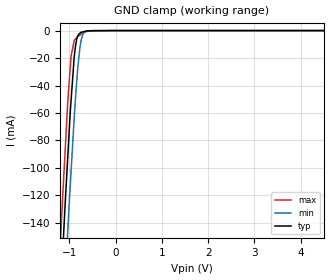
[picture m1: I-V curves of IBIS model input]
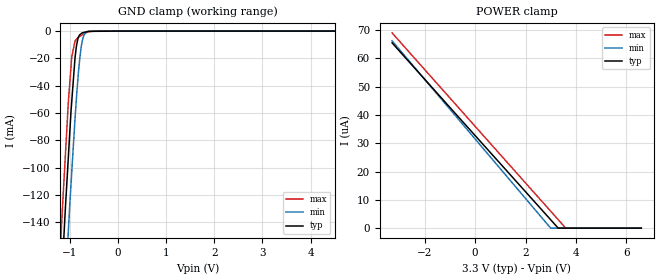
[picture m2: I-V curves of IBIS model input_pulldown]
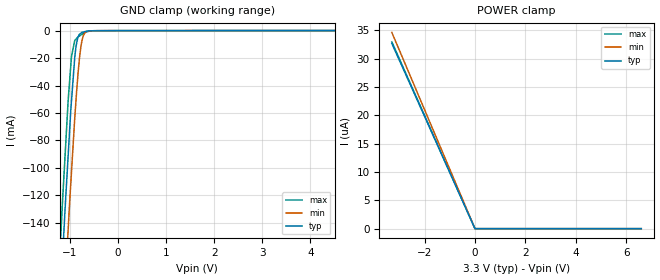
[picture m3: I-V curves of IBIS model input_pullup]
|Texas Instruments Incorporated
| Ultra-Small, Integrated Analog Front-End for Heart Rate Monitors and
| Low-Cost Pulse Oximeters
| Marketing part#   Digital Voltage Range   Package-type   #pins
| AFE4403   2.0V-3.6V   WCSP   36
[IBIS Ver]   4.1
[File name]   afe4403.ibs
[File Rev]   1.0
[Date]   6/3/2014
[Source]
| Texas Instruments Incorporated.
| Analog-eLab Design Center, HPA
| 12500 TI Blvd
| Dallas, TX -75243
[Notes]   Revision History:
| Rev 1.0: 6/3/2014
| - Initial version of the model
| - Model generated from simulations in TISPICE
| - Model matched to SPICE simulation
| - C_comp although listed in numerical order of value are
|   obtained from varying PVT conditions. For PVT conditions for
|   each specific value refer the buffer description under
|   respective [Model]. IBIS model user is responsible for using
|   appropriate C_comp to simulate for Signal Integrity.
| - All the models except io are taken from available IBIS model of AFE4490.
|*   EXCEPTION:   *
|*   - For input_pulldown and io models,there will be small leakage currents  *
|*   in POWER Clamp IV table because of a pulldown resistor R0 is connected *
|*   to PAD.   *
|*   - For model input_pullup,there will be  small leakage currents in GND   *
|*   Clamp IV table because of a pullup resistor R0 is connected to PAD.   *
[Disclaimer]
| This model is designed as an aid for customers of Texas Instruments.
| TI and its licensors and suppliers make no warranties, either expressed
| or implied, with respect to this  model, including the warranties of
| merchantability or fitness for a particular purpose. The model is
| provided solely on an "as is" basis. The entire risk as to its quality
| and performance is with the customer.
[Copyright]
(C) Copyright 2014 Texas Instruments Incorporated.All rights reserved.
|   AFE4403
[Component]   AFE4403
[Manufacturer]   TI
[Package]   |36 WCSP package
|   typ   min   max
R_pkg   0.01   0.008   0.12
L_pkg   0.1nH   0.08nH   0.12nH
C_pkg   0.1pF   0.08pF   0.12pF
[Pin]  signal_name   model_name   R_pin   L_pin   C_pin
A1   DNC   nc   na   na   na
A2   TX_CTRL_SUP   power   na   na   na
A3   LED_DRV_GND   gnd   na   na   na
A4   TXN   nc   na   na   na
A5   TXP   nc   na   na   na
A6   LED_DRV_SUP   power   na   na   na
B1   TX_REF   nc   na   na   na
B2   RX_DIG_GND   gnd   na   na   na
B3   TX3   nc   na   na   na
B4   DIAG_END   outp   na   na   na
B5   TG_EN   nc   na   na   na
B6   TG_OUT   io   na   na   na
C1   DNC   nc   na   na   na
C2   BG   nc   na   na   na
C3   AFE_PDN   input   na   na   na
C4   SPISIMO   outp   na   na   na
C5   SPISOMI   input_pulldown   na   na   na
C6   SCLK   input_pulldown   na   na   na
D1   VCM   nc   na   na   na
D2   VSS   gnd   na   na   na
D3   DNC   nc   na   na   na
D4   _RESET   input_pullup   na   na   na
D5   ADC_RDY   outp   na   na   na
D6   SPISTE   input_pullup   na   na   na
E1   INP   nc   na   na   na
E2   RX_ANA_GND   gnd   na   na   na
E3   DNC   nc   na   na   na
E4   RX_ANA_SUP   power   na   na   na
E5   RX_DIG_SUP   power   na   na   na
E6   CLKOUT   outp   na   na   na
F1   INN   nc   na   na   na
F2   RX_ANA_SUP   power   na   na   na
F3   XIN   nc   na   na   na
F4   XOUT   nc   na   na   na
F5   DNC   nc   na   na   na
F6   RX_DIG_GND   gnd   na   na   na
| Models and submodels in the file (5): input (Input), input_pulldown (Input), input_pullup (Input), outp (Output), io (I/O)
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|   input Model
[Model]   input
Model_type   Input
Vinl = 0.66
Vinh = 2.64
|   typ   min   max
|   (nom PVT)   (fast PVT)   (slow PVT)
C_comp   3.312e-13   3.289e-13   3.358e-13
[Model spec]
|subparameter
Vinl   0.66   0.6   0.72
Vinh   2.64   2.4   2.88
| Where nom  PVT is Nominal Process, 3.3V, 27C
|   Fast PVT is Strong Process,  3.6V, -40C
|   Slow PVT is Weak Process,   3V, 105C
[Voltage Range]   3.3   3   3.6
|Junction Temperature
[Temperature Range]   27   105   -40
[Power Clamp Reference]   3.3   3   3.6
[GND Clamp Reference]   0   0   0
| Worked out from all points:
|   GND clamp passes 1 mA (typ) near -0.72 V on its own axis
[GND Clamp]
|   Voltage   I(typ)   I(min)   I(max)
-3.3V     -1.734A    -1.762A    -1.725A
-1.27V    -245.7mA   -302.2mA   -207.4mA
-1.156V   -168.6mA   -223.4mA   -127.4mA
-1.137V   -156.2mA   -210.7mA   -115.7mA
-1.099V   -130.6mA   -186.4mA   -91.68mA
-1.037V   -92.87mA   -146.8mA   -52.56mA
-964.8mV  -51.35mA   -103.1mA   -18.88mA
-897.6mV  -19.84mA   -64.25mA   -7.375mA
-825mV    -4.345mA   -29.78mA   -4.502mA
-745.8mV  -1.232mA   -7.144mA   -2.676mA
-591mV    -190.8uA   -137.2uA   -416.9uA
6.6V      0A         0A         0A
[POWER Clamp]
|   Voltage   I(typ)   I(min)   I(max)
-3.3V     0A         0A         0A
0V        0A         0A         0A
6.6V      0A         0A         0A
|   input_pulldown Model
[Model]   input_pulldown
Model_type   Input
Vinl = 0.66
Vinh = 2.64
|   typ   min   max
|   (nom PVT)   (fast PVT)   (slow PVT)
C_comp   3.312e-13   3.289e-13   3.358e-13
[Model spec]
|subparameter
Vinl   0.66   0.6   0.72
Vinh   2.64   2.4   2.88
| Where nom  PVT is Nominal Process, 3.3V, 27C
|   Fast PVT is Strong Process,  3.6V, -40C
|   Slow PVT is Weak Process,   3V, 105C
[Voltage Range]   3.3   3   3.6
|Junction Temperature
[Temperature Range]   27   105   -40
[Power Clamp Reference]   3.3   3   3.6
[GND Clamp Reference]   0   0   0
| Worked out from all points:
|   GND clamp passes 1 mA (typ) near -0.72 V on its own axis
[GND Clamp]
|   Voltage   I(typ)   I(min)   I(max)
-3.3V     -1.734A    -1.762A    -1.725A
-1.27V    -245.7mA   -302.2mA   -207.4mA
-1.156V   -168.6mA   -223.4mA   -127.4mA
-1.137V   -156.2mA   -210.7mA   -115.7mA
-1.099V   -130.6mA   -186.4mA   -91.68mA
-1.037V   -92.87mA   -146.8mA   -52.57mA
-964.8mV  -51.35mA   -103.1mA   -18.88mA
-897.6mV  -19.84mA   -64.26mA   -7.379mA
-825mV    -4.348mA   -29.78mA   -4.505mA
-745.8mV  -1.237mA   -7.146mA   -2.68mA
-591mV    -195.8uA   -141.5uA   -421.6uA
6.6V      0A         0A         0A
[POWER Clamp]
|   Voltage   I(typ)   I(min)   I(max)
-3.3V     65.41uA    66.12uA    68.93uA
2.997V    3uA        31.46nA    6.017uA
3.297V    32.67nA    0A         3.027uA
3.604V    0A         0A         0A
6.6V      0A         0A         0A
|   input_pullup Model
[Model]   input_pullup
Model_type   Input
Vinl = 0.66
Vinh = 2.64
|   typ   min   max
|   (nom PVT)   (fast PVT)   (slow PVT)
C_comp   3.312e-13   3.289e-13   3.358e-13
[Model spec]
|subparameter
Vinl   0.66   0.6   0.72
Vinh   2.64   2.4   2.88
| Where nom  PVT is Nominal Process, 3.3V, 27C
|   Fast PVT is Strong Process,  3.6V, -40C
|   Slow PVT is Weak Process,   3V, 105C
[Voltage Range]   3.3   3   3.6
|Junction Temperature
[Temperature Range]   27   105   -40
[Power Clamp Reference]   3.3   3   3.6
[GND Clamp Reference]   0   0   0
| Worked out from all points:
|   GND clamp passes 1 mA (typ) near -0.71 V on its own axis
[GND Clamp]
|   Voltage   I(typ)   I(min)   I(max)
-3.3V     -1.734A    -1.762A    -1.725A
-1.27V    -245.7mA   -302.2mA   -207.4mA
-1.156V   -168.6mA   -223.4mA   -127.4mA
-1.137V   -156.2mA   -210.7mA   -115.7mA
-1.099V   -130.6mA   -186.4mA   -91.69mA
-1.037V   -92.88mA   -146.8mA   -52.58mA
-964.8mV  -51.36mA   -103.1mA   -18.9mA
-881.1mV  -14.53mA   -55.87mA   -6.602mA
-798mV    -2.701mA   -19.89mA   -3.904mA
-745.8mV  -1.258mA   -7.155mA   -2.702mA
-591mV    -235.2uA   -166.6uA   -451.7uA
6.6V      0A         0A         0A
[POWER Clamp]
|   Voltage   I(typ)   I(min)   I(max)
-3.3V     32.68uA    34.62uA    32.94uA
-1.911V   18.92uA    20.04uA    19.07uA
-33.83fV  0A         0A         0A
6.6V      0A         0A         0A
